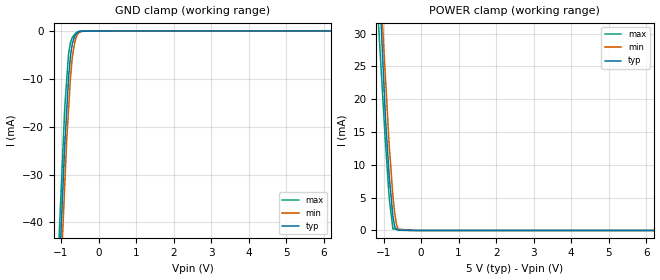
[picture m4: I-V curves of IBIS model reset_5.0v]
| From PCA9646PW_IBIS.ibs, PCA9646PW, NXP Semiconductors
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[Model] reset_5.0v
Model_type Input
Vinl = 900.000mV
Vinh = 4.80000V
C_comp 695.000fF 691.000fF 699.000fF
| variable typ   min   max
[Voltage Range] 5.00000V 4.50000V 5.50000V
[POWER Clamp Reference] 5.00000V 4.50000V 5.50000V
[GND Clamp Reference] 0.00000V 0.00000V 0.00000V
[Temperature Range]   25   85   -40
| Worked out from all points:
|   GND clamp passes 1 mA (typ) near -0.62 V on its own axis
|   POWER clamp passes 1 mA (typ) near -0.71 V on its own axis
[GND Clamp]
-5V       -769.3mA   -773.1mA   -750mA
-900mV    -23.68mA   -32.07mA   -15.91mA
-850mV    -16.78mA   -23.03mA   -10.38mA
-800mV    -9.872mA   -16.48mA   -4.856mA
-750mV    -5.327mA   -9.922mA   -2.468mA
-700mV    -2.633mA   -5.546mA   -1.35mA
-650mV    -1.363mA   -2.96mA    -865.5uA
-600mV    -657.7uA   -1.366mA   -380.9uA
-550mV    -296uA     -596.3uA   -141uA
-450mV    -89.66uA   -85.33uA   -29.3uA
-225mV    -7.223uA   -6.377uA   -516.8nA
10V       10.81uA    1.638uA    79.28uA
[POWER Clamp]
-5V       517.3mA    443.6mA    409.6mA
-1.25V    54.33mA    54.56mA    42.78mA
-950mV    17.29mA    23.43mA    13.43mA
-850mV    8.325mA    13.06mA    5.028mA
-750mV    2.183mA    5.224mA    235.9uA
-700mV    538uA      2.573mA    217uA
-650mV    106.2uA    762uA      198.1uA
-600mV    20.1uA     126uA      179.3uA
-100mV    0A         0A         0A
10V       0A         0A         0A
